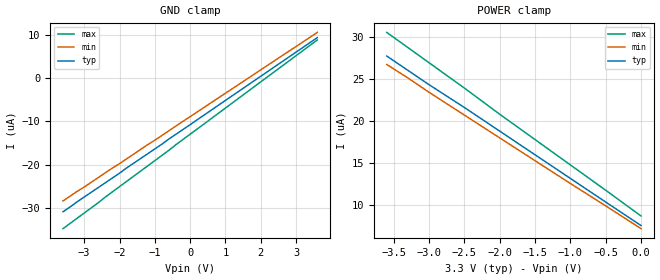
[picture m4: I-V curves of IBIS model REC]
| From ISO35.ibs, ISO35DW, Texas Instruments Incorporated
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|   Receiver Input / Model
[Model]   REC
Model_type   Input
|Signals   A,B
Vinh = 2.0
Vinl = 0.8
|   typ   min   max
C_comp   3.0pF   2.5pF   3.5pF
|   typ   min   max
[Temperature Range]   27   -40   85
[Voltage range]   3.3V   3.0V   3.6V
[GND_clamp]
|   Voltage   I(typ)   I(min)   I(max)
-3.6V     -30.9uA    -28.4uA    -34.8uA
-3.2V     -28.6uA    -26.2uA    -32.4uA
-2V       -22uA      -19.8uA    -25.1uA
3.6V      9.29uA     10.5uA     8.75uA
[Power_clamp]
| Note that the[POWER_clamp]voltage table is referenced to Vcc
| and is calculated using Vtable=Vcc - Vmeasured.
|   Voltage   I(typ)   I(min)   I(max)
-3.6V     27.7uA     26.7uA     30.5uA
-3.3V     26uA       25.1uA     28.7uA
-3V       24.3uA     23.4uA     26.9uA
-2.5V     21.6uA     20.7uA     23.9uA
-2V       18.8uA     18uA       20.8uA
-1.5V     16uA       15.3uA     17.8uA
-1V       13.2uA     12.6uA     14.8uA
-500mV    10.4uA     9.95uA     11.8uA
0V        7.62uA     7.25uA     8.75uA
